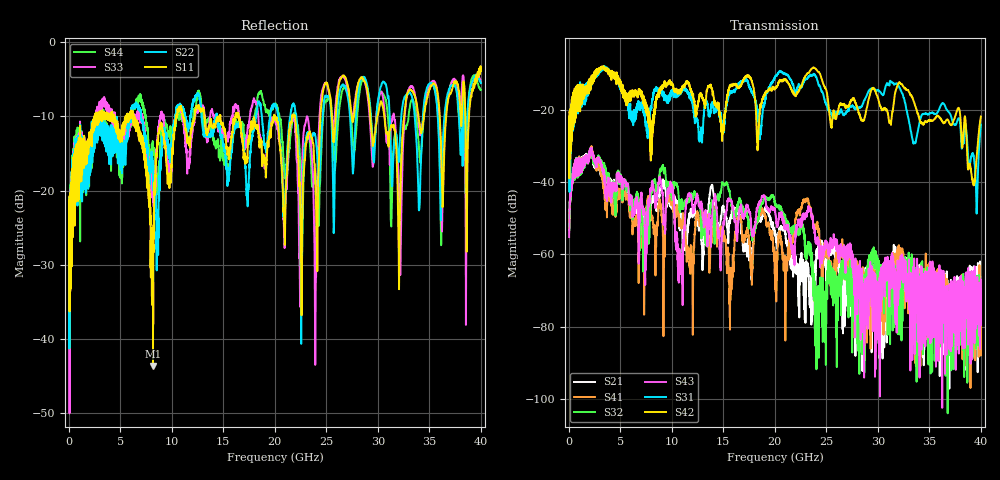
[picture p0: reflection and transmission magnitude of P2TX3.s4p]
!Agilent Technologies,N5245A,MY49151084,A.09.20.08
!Agilent N5245A: A.09.20.08
!Date: Thursday, March 01, 2012 14:46:06
!Correction: S11(Full 4 Port(1,2,3,4))
!S12(Full 4 Port(1,2,3,4))
!S13(Full 4 Port(1,2,3,4))
!S14(Full 4 Port(1,2,3,4))
!S21(Full 4 Port(1,2,3,4))
!S22(Full 4 Port(1,2,3,4))
!S23(Full 4 Port(1,2,3,4))
!S24(Full 4 Port(1,2,3,4))
!S31(Full 4 Port(1,2,3,4))
!S32(Full 4 Port(1,2,3,4))
!S33(Full 4 Port(1,2,3,4))
!S34(Full 4 Port(1,2,3,4))
!S41(Full 4 Port(1,2,3,4))
!S42(Full 4 Port(1,2,3,4))
!S43(Full 4 Port(1,2,3,4))
!S44(Full 4 Port(1,2,3,4))
!S4P File: Measurements: <S11,S12,S13,S14>,
!<S21,S22,S23,S24>,
!<S31,S32,S33,S34>,
!<S41,S42,S43,S44>:
# Hz S  dB  R 50
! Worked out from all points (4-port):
!   3996 points, 50 MHz to 40 GHz, reference 50 ohm
!   strongest paths, dB at 50 MHz, 10.04 GHz, 20.03 GHz, 30.02 GHz, 40 GHz:
!     S42: -25.0, -12.9, -14.2, -16.8, -21.9
!     S31: -25.6, -15.4, -10.9, -14.6, -24.1
!     S43: -55.3, -40.9, -48.3, -69.6, -67.0
!     S32: -51.8, -44.3, -45.9, -61.1, -73.7
!     S41: -51.5, -45.0, -62.0, -66.7, -69.4
!     S21: -51.4, -46.8, -53.5, -82.1, -68.8
!   lowest |S11| = -43.6 dB at 8.19 GHz (marker M1), VSWR 1.01, Z = 49.4 - j0.296 ohm
!   |S11| at or under -10 dB: start of sweep to 2.529 GHz; 6.361 GHz to 10.45 GHz (4.092 GHz wide, 48.7 % of centre); 16.51 GHz to 19.92 GHz (3.407 GHz wide, 18.7 % of centre)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
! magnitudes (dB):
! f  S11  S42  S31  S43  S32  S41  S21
! 50 MHz  -23.7  -25.0  -25.6  -55.3  -51.8  -51.5  -51.4
! 8.19 GHz  -43.6  -22.9  -16.6  -40.9  -39.9  -51.7  -44.0
! 10.89 GHz  -8.7  -15.3  -15.2  -64.5  -45.9  -52.2  -49.2
! 19.77 GHz  -11.0  -13.8  -12.4  -47.1  -44.2  -54.6  -52.0
! 24.06 GHz  -24.9  -9.1  -11.3  -56.7  -75.9  -52.4  -60.1
! 24.88 GHz  -5.6  -13.9  -18.0  -57.9  -84.4  -57.7  -61.7
! 40 GHz  -3.9  -21.9  -24.1  -67.0  -73.7  -69.4  -68.8
